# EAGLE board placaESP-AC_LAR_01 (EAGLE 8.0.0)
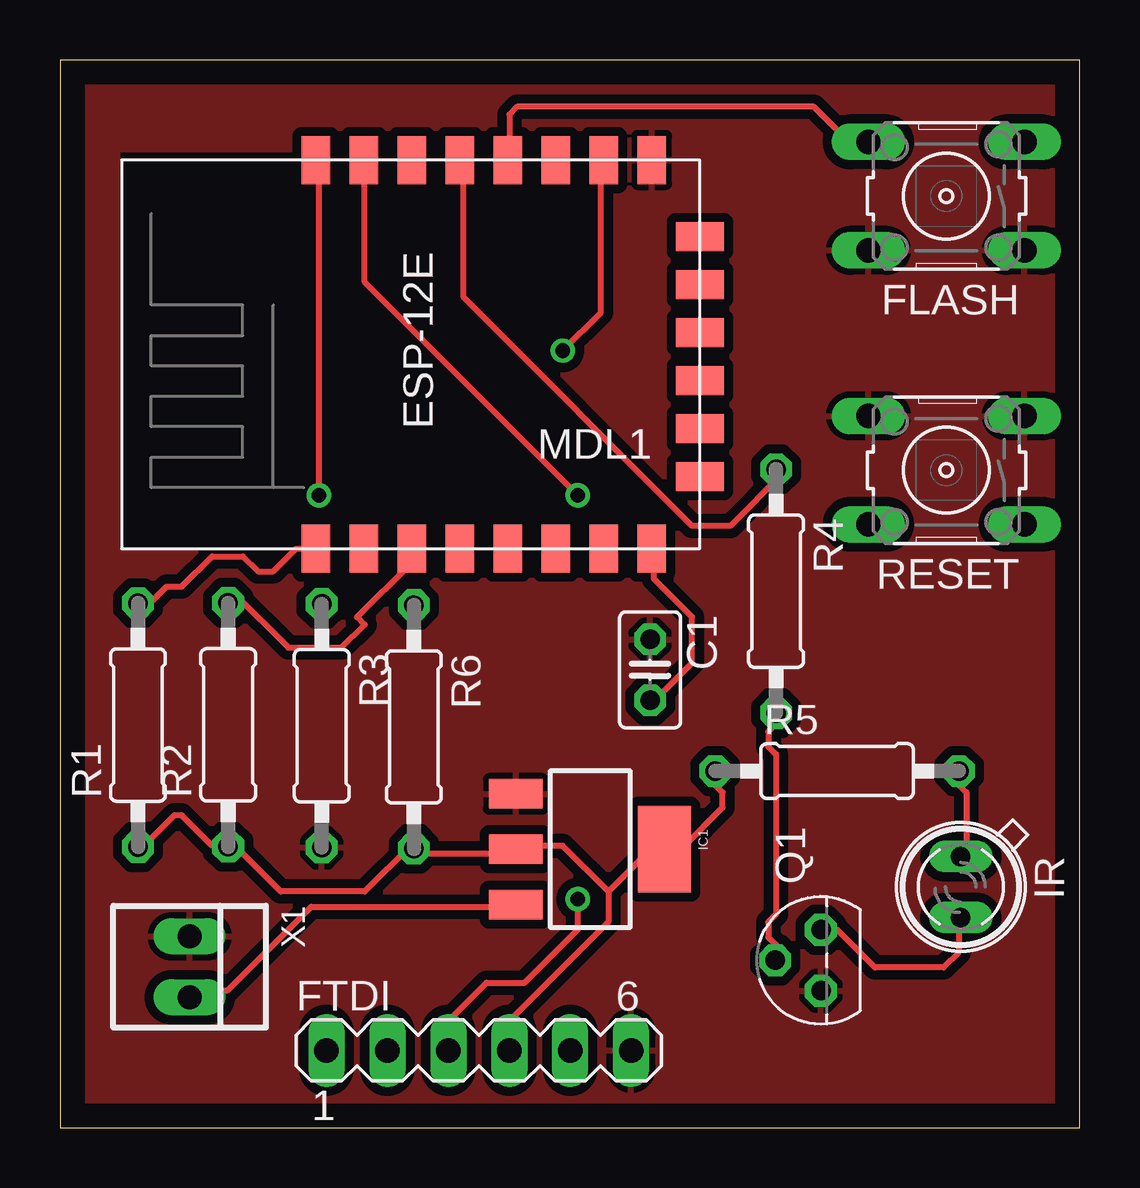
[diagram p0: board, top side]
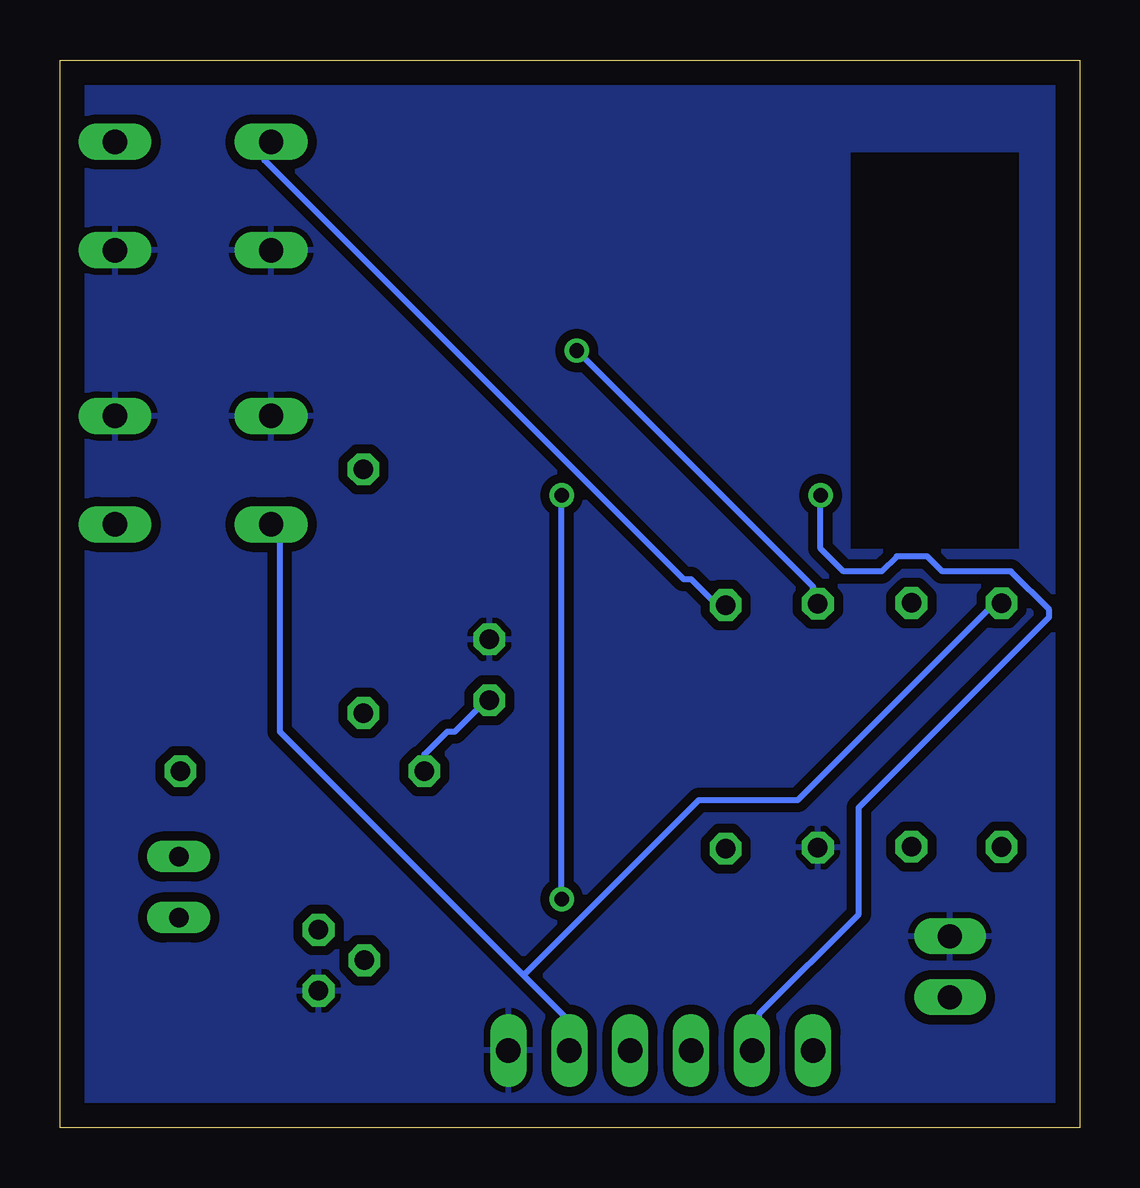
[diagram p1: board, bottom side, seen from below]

Size 42.5 x 44.5 mm. Coordinates in mm from the lower left corner, seen from the top.
Outline: 0,0 42.5,0 42.5,44.5 0,44.5 0,0
Copper layers (1*16): Top 0.035mm / dielectric 1.5mm / Bottom 0.035mm
Design rules "default *": minimum track width 10mil, minimum drill 24mil, track to track 15mil, track to pad 15mil, pad to pad 15mil, via to via 15mil, smd to smd 8mil, copper to edge 40mil, drill to drill 8mil, minimum pad ring 10mil, minimum via ring 8mil, stop-mask expansion 4mil, vias tented up to drill 0mil, thermal gap 10mil

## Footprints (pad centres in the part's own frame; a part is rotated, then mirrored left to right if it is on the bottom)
C025-025X050 = drill 0.813 octagon: 1 -1.27,0; 2 1.27,0
B3F-10XX = drill 1.016 long: 1 -3.251,2.261; 2 3.251,2.261; 3 -3.251,-2.261; 4 3.251,-2.261
MA06-1 = drill 1.016 long: 1 -6.35,0; 2 -3.81,0; 3 -1.27,0; 4 1.27,0; 5 3.81,0; 6 6.35,0
AMS1117 = smd 1.219 x 2.235: GND -2.311,-3.099; VIN 2.311,-3.099; VOUT 0,-3.099 | smd 3.6 x 2.2: HEATSINK 0,3.099
SFH482 = drill 0.813 long: A -1.27,0; K 1.27,0
ESP8266-ESP12E = smd 2 x 1.2: 1 -7.62,5.84; 2 -7.62,3.84; 3 -7.62,1.84; 4 -7.62,-0.16; 5 -7.62,-2.16; 6 -7.62,-4.16; 7 -7.62,-6.16; 8 -7.62,-8.16; 9 8.58,-8.16; 10 8.58,-6.16; 11 8.58,-4.16; 12 8.58,-2.16; 13 8.58,-0.16; 14 8.58,1.84; 15 8.58,3.84; 16 8.58,5.84 | smd 1.2 x 2: 17 -4.62,-10.16; 18 -2.62,-10.16; 19 -0.62,-10.16; 20 1.38,-10.16; 21 3.38,-10.16; 22 5.38,-10.16
TO92 = drill 0.813 octagon: 1 1.27,0; 2 0,1.905; 3 -1.27,0
0207/10 = drill 0.813 octagon: 1 -5.08,0; 2 5.08,0
22-23-2021 = drill 1 long: 1 -1.27,0; 2 1.27,0

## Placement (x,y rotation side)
C1  100n  [C025-025X050]  24.6,19.08 270 top
FLASH  [B3F-10XX]  36.95,38.83 180 top
FTDI  [MA06-1]  17.46,3.21 0 top
IC1  [AMS1117]  22.1,11.6 270 top
IR  [SFH482]  37.55,10.03 270 top
MDL1  [ESP8266-ESP12E]  16.51,31.75 90 top
Q1  2N4401  [TO92]  31.72,6.97 90 top
R1  10k  [0207/10]  3.25,16.78 90 top
R2  10k  [0207/10]  7.01,16.79 90 top
R3  10k  [0207/10]  10.91,16.75 270 top
R4  4k7  [0207/10]  29.85,22.36 270 top
R5  100R  [0207/10]  32.39,14.86 0 top
R6  10k  [0207/10]  14.75,16.7 270 top
RESET  [B3F-10XX]  36.95,27.4 180 top
X1  22-23-2021  [22-23-2021]  5.4,6.7 270 top

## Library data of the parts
C1 R1-R6 = rcl
FLASH RESET = switch-omron; MPN: B3F-1000; OC_FARNELL: 176432; OC_NEWARK: 36M3542
FTDI = con-lstb; OC_FARNELL: unknown; OC_NEWARK: unknown
IC1 = kaibader
IR = led
MDL1 = ESP8266-ESP12E
Q1 = transistor-npn
X1 = con-molex; MF: MOLEX; MPN: 22-23-2021; OC_FARNELL: 1462926; OC_NEWARK: 25C3832

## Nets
CTS: FTDI.5 MDL1.1 R1.2 RESET.2
DTR: FTDI.1
GND: C1.1 FLASH.1 FLASH.2 FTDI.6 IC1.GND MDL1.9 Q1.3 R3.2 RESET.3 RESET.4 X1.1
IN+: IC1.VIN X1.2
IO4: MDL1.13 R4.1
N$1: MDL1.3 R2.2
N$2: IR.A R5.2
N$3: Q1.2 R4.2
N$4: IR.K Q1.1
N$5: MDL1.10 R3.1
N$6: FLASH.4 MDL1.12 R6.1
RXI: FTDI.2 MDL1.16
TXO: FTDI.3 MDL1.15
VCC: C1.2 FTDI.4 IC1.HEATSINK IC1.VOUT MDL1.8 R1.1 R2.1 R5.1 R6.2

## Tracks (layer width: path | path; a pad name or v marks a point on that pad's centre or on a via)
CTS
  Top 0.254: MDL1.1 9.84,24.13 8.89,23.18 8.26,23.18 7.62,23.81 6.35,23.81 5.08,22.54 4.45,22.54 3.49,21.59 R1.2
  Bottom 0.254: 23.18,6.35 33.34,16.51 33.34,24.77 33.66,25.08 RESET.2 | 23.18,6.35 21.27,4.45 21.27,3.49 FTDI.5 | 23.18,6.35 15.88,13.65 11.75,13.65 3.81,21.59 3.49,21.59 R1.2
GND
  pour Bottom: 0,0 0,44.5 42.5,44.5 42.5,0
  pour Top: 0,0 42.5,0 42.5,44.5 0,44.5
IN+
  Top 0.254: IC1.VIN 18.73,9.21 10.48,9.21 6.99,5.71 5.71,5.71 X1.2
IO4
  Top 0.254: MDL1.13 16.83,40.32 16.83,34.61 26.35,25.08 27.94,25.08 30.16,27.3 R4.1
N$1
  Top 0.254: MDL1.3 14.61,24.13 14.61,23.5 12.38,21.27 12.7,20.95 11.75,20 9.53,20 7.3,22.23 6.99,21.91 R2.2
N$2
  Top 0.254: IR.A 37.78,11.43 37.78,13.97 37.15,14.61 37.47,14.92 R5.2
N$3
  Top 0.254: Q1.2 29.84,6.99 29.84,7.62 29.53,7.94 29.53,8.57 29.84,8.89 29.84,15.56 29.53,15.88 29.53,16.51 30.16,17.14 R4.2
N$4
  Top 0.254: Q1.1 31.75,8.26 32.38,8.26 33.97,6.67 36.83,6.67 37.47,7.3 37.47,8.57 IR.K
N$5  (via drill 0.61)
  Top 0.254: v20.95,32.38 22.54,33.97 22.54,40.32 MDL1.10
  Bottom 0.254: v20.95,32.38 11.11,22.54 11.11,21.91 R3.1
N$6
  Top 0.254: MDL1.12 18.73,40.64 18.73,42.23 19.05,42.55 31.43,42.55 32.7,41.27 33.66,41.27 FLASH.4
  Bottom 0.254: R6.1 14.92,21.91 15.24,21.91 16.19,22.86 16.51,22.86 33.97,40.32 33.97,40.96 FLASH.4
RXI  (via drill 0.61)
  Top 0.254: v10.79,26.35 10.79,40.32 MDL1.16
  Bottom 0.254: v10.79,26.35 10.79,24.13 9.84,23.18 8.26,23.18 7.62,23.81 6.35,23.81 5.71,23.18 2.86,23.18 1.27,21.59 1.27,21.27 9.21,13.34 9.21,8.89 13.34,4.76 13.34,3.49 FTDI.2
TXO  (via drill 0.61)
  Top 0.254: v21.59,26.35 12.7,35.24 12.7,40.32 MDL1.15 | v21.59,9.53 21.59,8.26 19.37,6.03 17.78,6.03 16.19,4.45 16.19,3.49 FTDI.3
  Bottom 0.254: v21.59,9.53 v21.59,26.35
VCC
  Top 0.254: R1.1 3.49,11.75 4.76,13.02 5.08,13.02 6.35,11.75 6.99,11.75 R2.1 7.3,11.43 7.62,11.43 9.21,9.84 12.7,9.84 14.61,11.75 R6.2 14.92,11.43 18.73,11.43 IC1.VOUT 19.05,11.75 20.95,11.75 22.86,9.84 | MDL1.8 24.77,24.13 24.77,22.86 26.35,21.27 26.35,19.37 25.08,18.1 25.08,17.78 24.77,17.78 C1.2 | R5.1 27.3,14.61 27.3,14.29 27.62,13.97 27.62,13.34 26.04,11.75 25.4,11.75 IC1.HEATSINK 25.08,11.43 24.45,11.43 22.86,9.84 | 22.86,9.84 22.86,8.57 18.73,4.45 18.73,3.49 FTDI.4
  Bottom 0.254: C1.2 24.77,17.78 26.04,16.51 26.35,16.51 27.3,15.56 27.3,14.92 R5.1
